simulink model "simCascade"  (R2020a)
settings: Solver=ode15s  StartTime=0.0  StopTime=tsim  MaxStep=1  RelTol=1e-3
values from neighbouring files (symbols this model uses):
  dQ1 = Q10-0.1*Q10    (= 1504.8)    [runTransformations.m]
  dQ2 = Q20+0    (= 836)    [runTransformations.m]
  dT0 = T00+0    (= 10)    [runTransformations.m]
  dv2 = v20+0    (= 0)    [runTransformations.m]    (also in FcOL.m = -0.391; runTransfOL.m = -1)
  KcC = 0    [runTransformations.m]
  nd = 2    [runTransformations.m]    (also in Main.m = size(d0,2); Main_OL.m = size(d0,2); runTestCalcBlk.m = size(d0,2); runTransf.m = size(d0,2))
  np = length(p)    [runTransformations.m]    (also in runH2Psim.m = length(param); Main.m = size(p,2); Main_OL.m = size(p,2); runTestCalcBlk.m = size(p,2))
  nu = 1    [runTransformations.m]    (also in runH2Psim.m = length(u0); Main.m; Main_OL.m; runTestCalcBlk.m)
  nx = 2    [runTransformations.m]    (also in H2P_Turbine_driven.m = param(end); runTD.m = length(x0); H2P_Boiler_driven.m = param(end); runBD.m = length(x0))
  p = [p;tau01;tau02]    [runTransformations.m]    (also in Main.m = [N, Fc0, rhoc, rhoh,U,A,cpc,cph]; Main_OL.m = [N, Fc0, rhoc, rhoh,U,A,cpc,cph]; runTestCalcBlk.m = [N, Fc0, rhoc, rhoh,U,A,cpc,cph]; NonlinearMap.m = [U;A;Fc(i);Fh;cpc;cph;Tcin;Thin])
  Q10 = -F*cp*(T00-T10)    (= 1672)    [runTransformations.m]
  Q20 = -F*cp*(T10-T20)    (= 836)    [runTransformations.m]
  T00 = 10    [runTransformations.m]
  tauIC = 1    [runTransformations.m]
  tdQ2 = 10    [runTransformations.m]
  tdT0 = 10    [runTransformations.m]
  tQ1 = 100    [runTransformations.m]
  tsp = 10    [runTransformations.m]
  v20 = 0    [runTransformations.m]    (also in runTransfOL.m = v00)
  x0 = [T10;T20]    [runTransformations.m]    (also in runTD.m = [TE0;TD0;TSh0;MD0; MSh0;w0;TA0;0;0;0;0;0;0;0;0;0]; runBD.m = [TE0;TD0;TSh0;MD0; MSh0;w0;TA0;0;0;0;0;0;0;0;0;0]; runFP.m = [TE0;TD0;TSh0;MD0; MSh0;w0;TA0;0;0;0;0;0;0;0]; runFPV2.m = [TE0;TD0;TSh0;MD0; MSh0;w0;TA0;0;0;0;0;0;0;0])
undefined symbols (not defined in the file or in its folder): Calc_v2, TanksODE

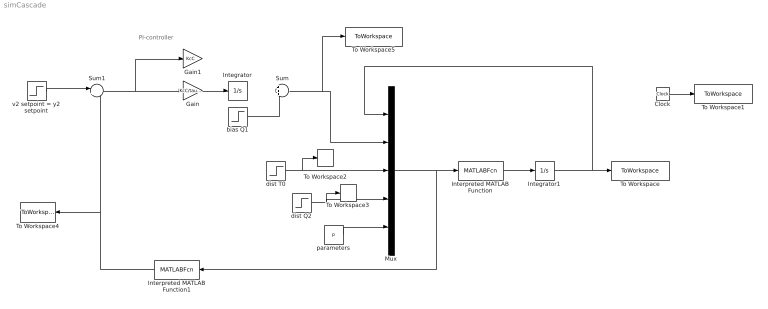
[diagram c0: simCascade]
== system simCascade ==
  note: PI-controller
  Clock : Clock
  Gain : Gain  Gain=KcC/tauIC  Multiplication=Matrix(K*u)
  Gain1 : Gain  Gain=KcC  Multiplication=Matrix(K*u)
  Integrator : Integrator
  Integrator1 : Integrator  InitialCondition=x0
  Interpreted MATLAB Function : MATLABFcn  MATLABFcn=TanksODE(u(1:nx),u(nx+1:nx+nu), u(nx+nu+1:nx+nu+nd), u(nx+nu+nd+1:nx+nu+nd+np))
  Interpreted MATLAB Function1 : MATLABFcn  MATLABFcn=Calc_v2(u(1:nx),u(nx+1:nx+nu), u(nx+nu+1:nx+nu+nd),u(nx+nu+nd+1:nx+nu+nd+np))
  Mux : Mux  Inputs=5
  Sum : Sum  Inputs=+++
  Sum1 : Sum  Inputs=|+-
  To Workspace : ToWorkspace  VariableName=y  SampleTime=-1
  To Workspace1 : ToWorkspace  VariableName=time  SampleTime=-1
  To Workspace2 : ToWorkspace  VariableName=T0  SampleTime=-1
  To Workspace3 : ToWorkspace  VariableName=Q2  SampleTime=-1
  To Workspace4 : ToWorkspace  VariableName=v2  SampleTime=-1
  To Workspace5 : ToWorkspace  VariableName=Q1  SampleTime=-1
  bias Q1 : Step  Time=tQ1  Before=Q10  After=dQ1  SampleTime=0
  dist Q2 : Step  Time=tdQ2  Before=Q20  After=dQ2  SampleTime=0
  dist T0 : Step  Time=tdT0  Before=T00  After=dT0  SampleTime=0
  parameters : Constant  Value=p
  v2 setpoint = y2 setpoint : Step  Time=tsp  Before=v20  After=dv2  SampleTime=0
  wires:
  Interpreted MATLAB Function/1 -> Integrator1/1
  Mux/1 -> Interpreted MATLAB Function1/1, Interpreted MATLAB Function/1
  parameters/1 -> Mux/5
  dist Q2/1 -> Mux/4, To Workspace3/1
  dist T0/1 -> To Workspace2/1, Mux/3
  Clock/1 -> To Workspace1/1
  Gain/1 -> Integrator/1
  Integrator/1 -> ?
  Sum/1 -> To Workspace5/1, Mux/2
  bias Q1/1 -> Sum/3
  Gain1/1 -> ?
  Sum1/1 -> Gain1/1, Gain/1
  v2 setpoint = y2 setpoint/1 -> Sum1/1
  Interpreted MATLAB Function1/1 -> Sum1/2, To Workspace4/1
  Integrator1/1 -> To Workspace/1, Mux/1
